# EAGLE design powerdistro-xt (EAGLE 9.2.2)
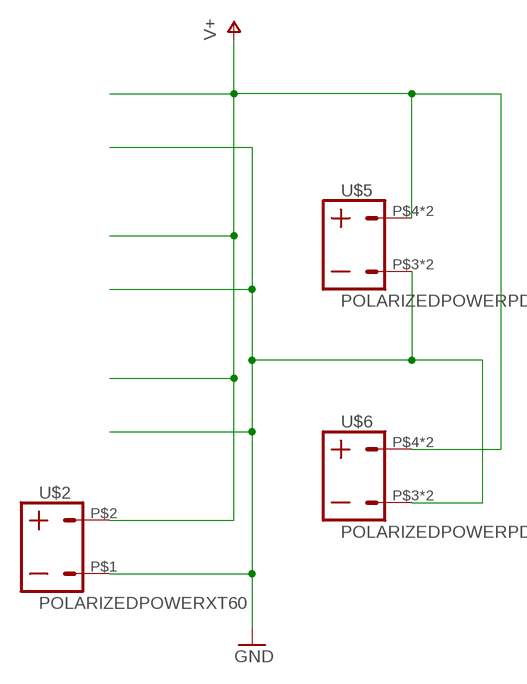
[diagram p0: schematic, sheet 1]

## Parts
U$2  POLARIZEDPOWERXT60  [XT60]
U$5  POLARIZEDPOWERPDB  [PDBCONN]
U$6  POLARIZEDPOWERPDB  [PDBCONN]

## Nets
GND: U$2.P$1 U$5.P$3 U$5.P$6 U$6.P$3 U$6.P$6
V+: U$2.P$2 U$5.P$4 U$5.P$5 U$6.P$4 U$6.P$5

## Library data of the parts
U$2 U$5 U$6 = connector:POLARIZEDPOWER

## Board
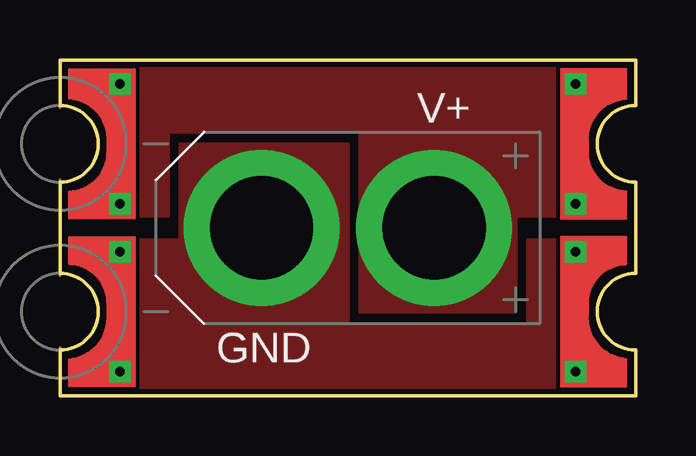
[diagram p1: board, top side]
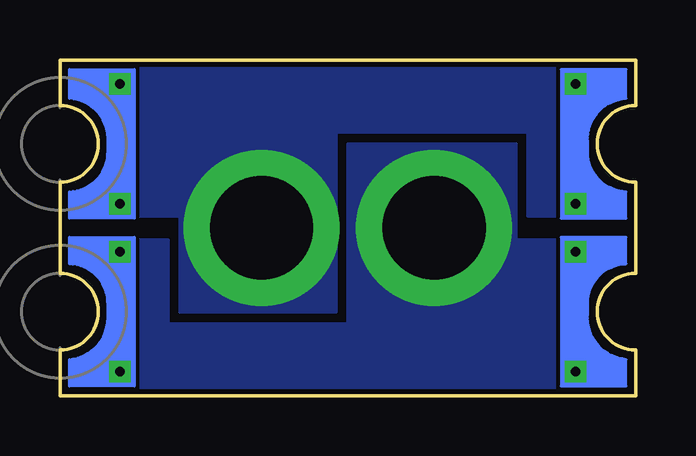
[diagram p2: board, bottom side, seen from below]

Size 24 x 14 mm. Coordinates in mm from the lower left corner, seen from the top.
Outline: 0,5.1 0,8.9 arc90 1.6,10.5 arc90 0,12.1 0,14 24,14 24,12.1 arc90 22.4,10.5 arc90 24,8.9 24,5.1 arc90 22.4,3.5 arc90 24,1.9 24,0 0,0 0,1.9 arc90 1.6,3.5 arc90 0,5.1
Copper layers (1*16): Top 0.035mm / dielectric 1.5mm / Bottom 0.035mm
Design rules "default *": minimum track width 6mil, minimum drill 0.35mm, track to track 6mil, track to pad 6mil, pad to pad 6mil, via to via 6mil, smd to smd 6mil, copper to edge 8mil, drill to drill 6mil, minimum pad ring 10mil, minimum via ring 8mil, stop-mask expansion 4mil, vias tented up to drill 0mil, thermal gap 10mil

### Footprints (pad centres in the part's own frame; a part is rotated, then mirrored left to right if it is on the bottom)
XT60 = drill 4.3 pad 6.5: P$1 3.6,0; P$2 -3.6,0
PDBCONN = drill 0.4 square: P$3 2.5,2.5; P$4 2.5,4.5; P$5 2.5,9.5; P$6 2.5,-2.5

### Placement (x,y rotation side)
U$2  12,7 180 top
U$5  0,3.5 0 top
U$6  24,3.5 0 bottom

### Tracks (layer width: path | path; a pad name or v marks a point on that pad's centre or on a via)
GND
  pour Top: -1,6.5 5,6.5 5,10.5 12,10.5 12,3 19.5,3 19.5,6.5 26.5,6.5 26.5,-0.5 -1,-0.5
  pour Bottom: -1.5,6.5 5,6.5 5,10.5 12,10.5 12,3 19.5,3 19.5,6.5 27,6.5 27,-1 -1.5,-1
V+
  pour Top: -1,7.5 4.5,7.5 4.5,11 12.5,11 12.5,3.5 19,3.5 19,7.5 26.5,7.5 26.5,15 -1,15
  pour Bottom: -1.5,7.5 4.5,7.5 4.5,11 12.5,11 12.5,3.5 19,3.5 19,7.5 27,7.5 27,15.5 -1.5,15.5

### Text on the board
tPlace: V+ | GND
